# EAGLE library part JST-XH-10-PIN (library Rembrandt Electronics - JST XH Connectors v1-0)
JST XH Connector 2 Pin Wire to board connector. Pitch: 2,54 mm, (0.100") Number of pins: 10 Created by Rembrandt Electronics www.rembrandtelectronics.com
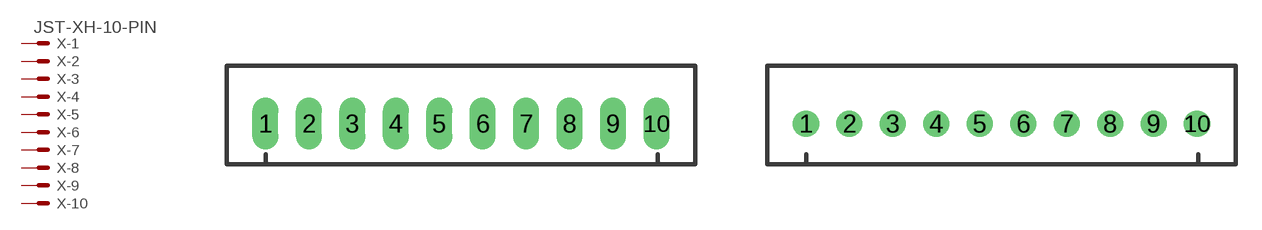
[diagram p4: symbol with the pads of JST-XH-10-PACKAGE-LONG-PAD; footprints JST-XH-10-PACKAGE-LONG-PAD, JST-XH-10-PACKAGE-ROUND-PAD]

Designator prefix X; gates -1=MV -2=M -3=M -4=M -5=M -6=M -7=M -8=M -9=M -10=M

## JST-XH-10-PIN-LONG-PAD  [JST-XH-10-PACKAGE-LONG-PAD]
1  -1:S  pas
2  -2:S  pas
3  -3:S  pas
4  -4:S  pas
5  -5:S  pas
6  -6:S  pas
7  -7:S  pas
8  -8:S  pas
9  -9:S  pas
10  -10:S  pas

## JST-XH-10-PIN-ROUND-PAD  [JST-XH-10-PACKAGE-ROUND-PAD]
Pads as for JST-XH-10-PACKAGE-LONG-PAD

## Footprint JST-XH-10-PACKAGE-LONG-PAD (pad centres in mm)
JST XH Connector Long Pads (Package) Wire to board connector. Pitch: 2,54 mm, (0.100") Number of pins: 10 Created by Rembrandt Electronics www.rembrandtelectronics.com
drill 1.016 long: 1 -11.43,0; 2 -8.89,0; 3 -6.35,0; 4 -3.81,0; 5 -1.27,0; 6 1.27,0; 7 3.81,0; 8 6.35,0; 9 8.89,0; 10 11.43,0

## Footprint JST-XH-10-PACKAGE-ROUND-PAD (pad centres in mm)
JST XH Connector Round Pads (Package) Wire to board connector. Pitch: 2,54 mm, (0.100") Number of pins: 10 Created by Rembrandt Electronics www.rembrandtelectronics.com
drill 1.016: 1 -11.43,0; 2 -8.89,0; 3 -6.35,0; 4 -3.81,0; 5 -1.27,0; 6 1.27,0; 7 3.81,0; 8 6.35,0; 9 8.89,0; 10 11.43,0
